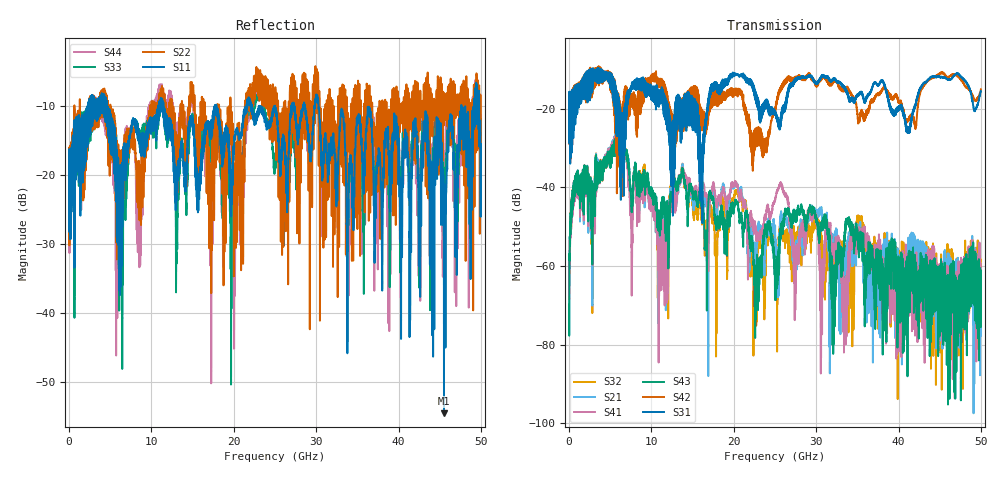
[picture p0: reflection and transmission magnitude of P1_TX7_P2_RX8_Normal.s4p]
!Keysight Technologies,N5225B,MY57041031,A.13.20.10
!Date: Friday, May 31, 2019 11:40:45
!Correction: S11(Full 4 Port(1,2,3,4))
!S12(Full 4 Port(1,2,3,4))
!S13(Full 4 Port(1,2,3,4))
!S14(Full 4 Port(1,2,3,4))
!S21(Full 4 Port(1,2,3,4))
!S22(Full 4 Port(1,2,3,4))
!S23(Full 4 Port(1,2,3,4))
!S24(Full 4 Port(1,2,3,4))
!S31(Full 4 Port(1,2,3,4))
!S32(Full 4 Port(1,2,3,4))
!S33(Full 4 Port(1,2,3,4))
!S34(Full 4 Port(1,2,3,4))
!S41(Full 4 Port(1,2,3,4))
!S42(Full 4 Port(1,2,3,4))
!S43(Full 4 Port(1,2,3,4))
!S44(Full 4 Port(1,2,3,4))
!S4P File: Measurements: <S11,S12,S13,S14>,
!<S21,S22,S23,S24>,
!<S31,S32,S33,S34>,
!<S41,S42,S43,S44>:
# Hz S  dB  R 50.0
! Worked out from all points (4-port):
!   5000 points, 10 MHz to 50 GHz, reference 50 ohm
!   strongest paths, dB at 10 MHz, 12.51 GHz, 25.01 GHz, 37.51 GHz, 50 GHz:
!     S31: -19.3, -39.1, -20.9, -14.0, -15.6
!     S42: -19.7, -22.3, -20.2, -16.4, -15.1
!     S43: -69.8, -42.1, -68.4, -57.7, -75.4
!     S41: -59.4, -44.1, -43.2, -54.8, -61.8
!     S21: -70.7, -43.1, -51.2, -59.2, -66.2
!     S32: -60.1, -41.1, -54.3, -76.0, -58.3
!   lowest |S11| = -54.5 dB at 45.52 GHz (marker M1), VSWR 1.00, Z = 49.9 + j0.177 ohm
!   |S11| at or under -10 dB: 4.613 GHz to 10.86 GHz (6.246 GHz wide, 80.7 % of centre); 11.46 GHz to 17.73 GHz (6.278 GHz wide, 43 % of centre); 30.28 GHz to 47.61 GHz (17.32 GHz wide, 44.5 % of centre)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
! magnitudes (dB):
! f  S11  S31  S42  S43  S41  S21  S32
! 10 MHz  -19.1  -19.3  -19.7  -69.8  -59.4  -70.7  -60.1
! 6.24 GHz  -20.4  -39.8  -24.9  -27.1  -26.8  -26.6  -26.9
! 10.92 GHz  -10.7  -15.4  -13.7  -49.7  -60.0  -63.0  -63.7
! 25.65 GHz  -19.0  -23.1  -15.3  -51.0  -38.9  -47.3  -51.1
! 33.46 GHz  -14.0  -15.0  -14.9  -51.3  -77.7  -62.3  -58.6
! 45.52 GHz  -54.5  -12.0  -11.1  -63.8  -69.9  -58.1  -65.7
! 50 GHz  -15.5  -15.6  -15.1  -75.4  -61.8  -66.2  -58.3
